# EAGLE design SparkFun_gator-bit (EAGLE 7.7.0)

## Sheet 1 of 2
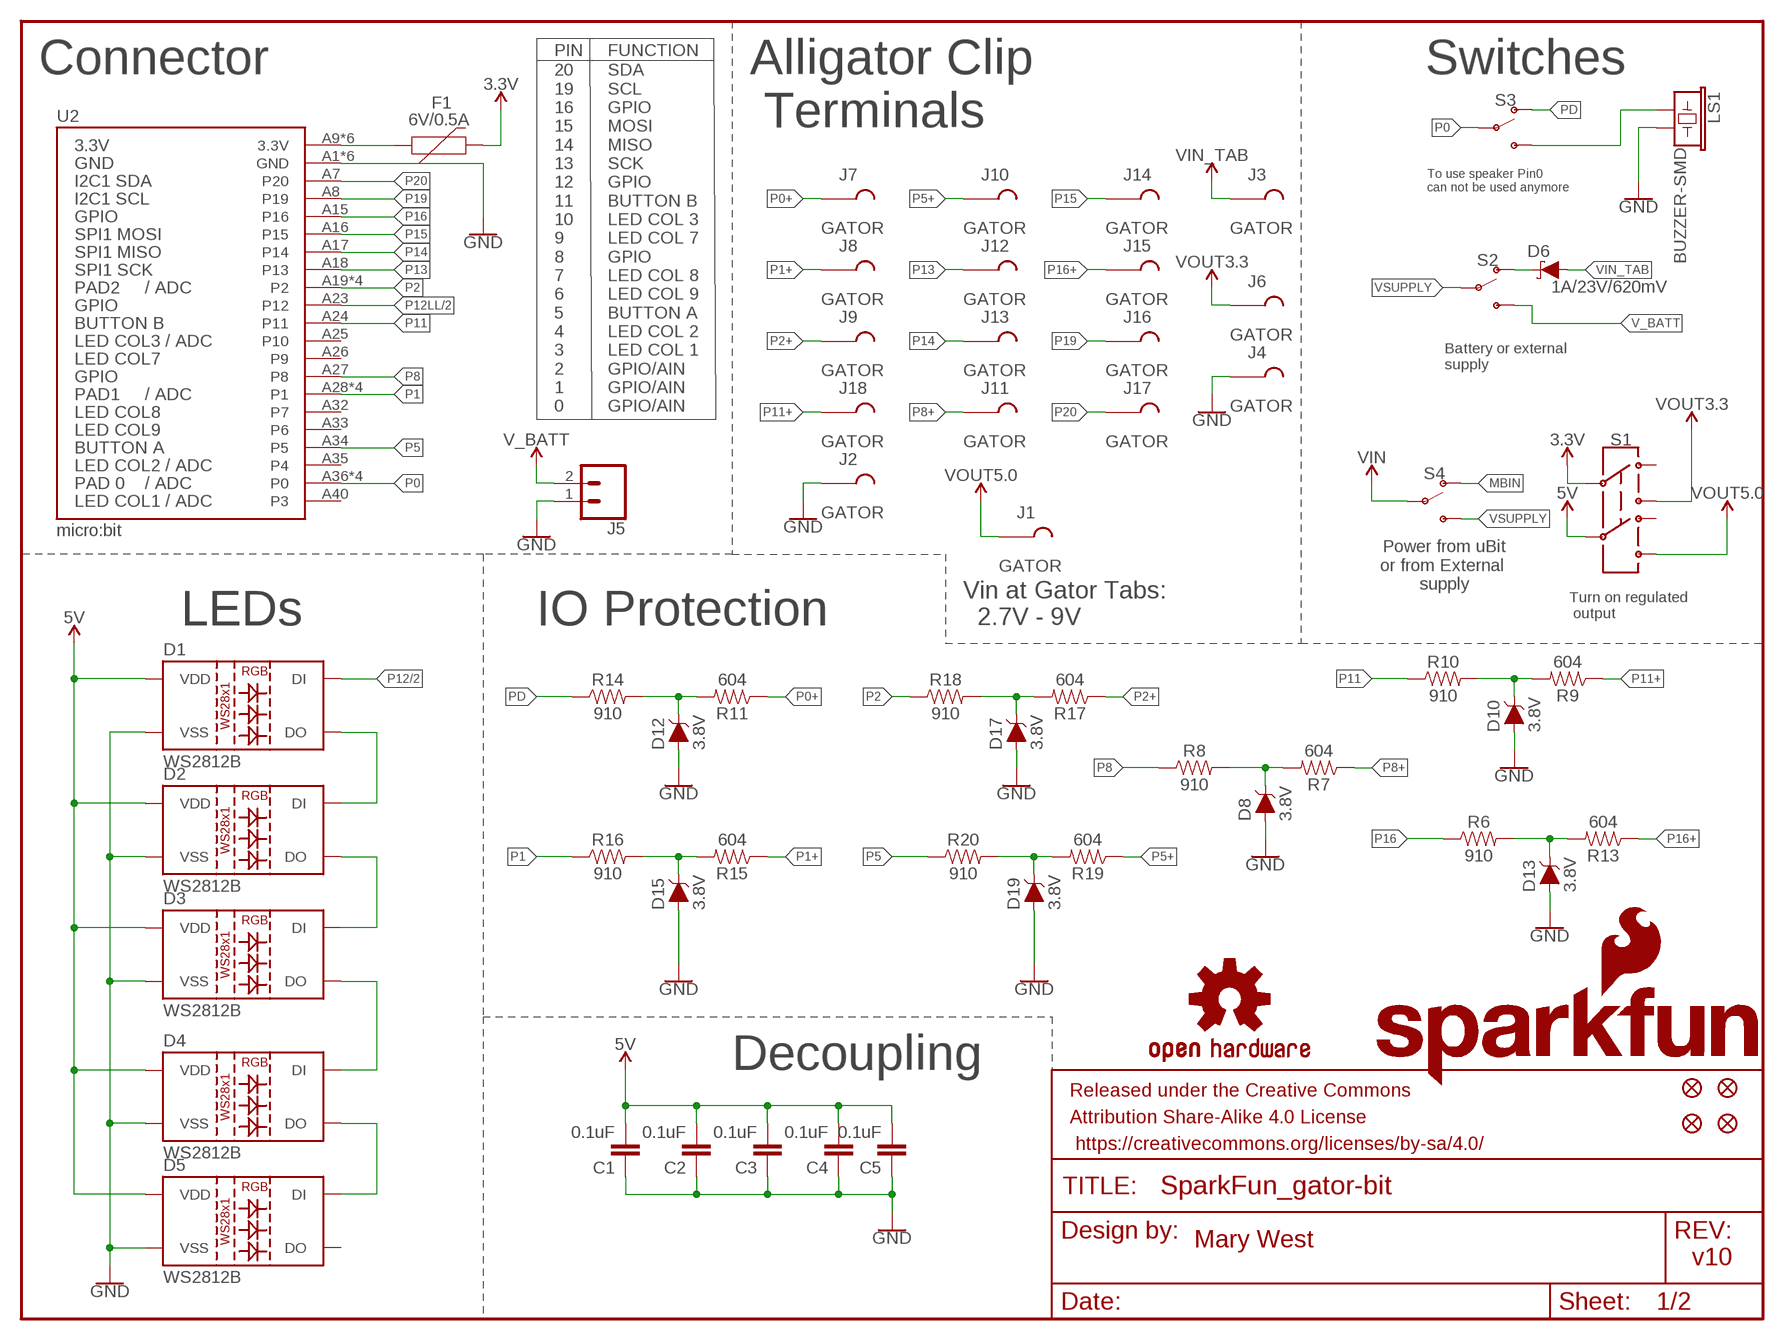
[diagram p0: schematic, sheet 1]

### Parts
C1  0.1uF  0.1UF-0603-25V-(+80/-20%)  [0603]
C2  0.1uF  0.1UF-0603-25V-(+80/-20%)  [0603]
C3  0.1uF  0.1UF-0603-25V-(+80/-20%)  [0603]
C4  0.1uF  0.1UF-0603-25V-(+80/-20%)  [0603]
C5  0.1uF  0.1UF-0603-25V-(+80/-20%)  [0603]
D1  WS2812B  [WS2812B]
D2  WS2812B  [WS2812B]
D3  WS2812B  [WS2812B]
D4  WS2812B  [WS2812B]
D5  WS2812B  [WS2812B]
D6  1A/23V/620mV  DIODE-SCHOTTKY-BAT20J  [SOD-323]
D8  3.8V  PDZVTR3.6B  [SOD-128]
D10  3.8V  PDZVTR3.6B  [SOD-128]
D12  3.8V  PDZVTR3.6B  [SOD-128]
D13  3.8V  PDZVTR3.6B  [SOD-128]
D15  3.8V  PDZVTR3.6B  [SOD-128]
D17  3.8V  PDZVTR3.6B  [SOD-128]
D19  3.8V  PDZVTR3.6B  [SOD-128]
F1  6V/0.5A  PPTC_HALF-AMP  [1206]
FD1  FIDUCIAL1X2  [FIDUCIAL-1X2]
FD2  FIDUCIAL1X2  [FIDUCIAL-1X2]
FD3  FIDUCIAL1X2  [FIDUCIAL-1X2]
FD4  FIDUCIAL1X2  [FIDUCIAL-1X2]
FRAME1  FRAME-LETTER  [CREATIVE_COMMONS]
J1  GATOR  [GATOR]
J2  GATOR  [GATOR]
J3  GATOR  [GATOR]
J4  GATOR  [GATOR]
J5  CONN_02-JST-2MM-SMT  [JST-2-SMD]
J6  GATOR  [GATOR]
J7  GATOR  [GATOR]
J8  GATOR  [GATOR]
J9  GATOR  [GATOR]
J10  GATOR  [GATOR]
J11  GATOR  [GATOR]
J12  GATOR  [GATOR]
J13  GATOR  [GATOR]
J14  GATOR  [GATOR]
J15  GATOR  [GATOR]
J16  GATOR  [GATOR]
J17  GATOR  [GATOR]
J18  GATOR  [GATOR]
LOGO1  SFE_LOGO_NAME_FLAME.3_INCH  [SFE_LOGO_NAME_FLAME_.3]
LOGO2  OSHW-LOGOM  [OSHW-LOGO-M]
LS1  BUZZER-SMD  [BUZZER-CCV]
R6  910  910OHMOHMS-0603-1/10W-1%  [0603]
R7  604  604OHMOHMS-0603-1/10W-1%  [0603]
R8  910  910OHMOHMS-0603-1/10W-1%  [0603]
R9  604  604OHMOHMS-0603-1/10W-1%  [0603]
R10  910  910OHMOHMS-0603-1/10W-1%  [0603]
R11  604  604OHMOHMS-0603-1/10W-1%  [0603]
R13  604  604OHMOHMS-0603-1/10W-1%  [0603]
R14  910  910OHMOHMS-0603-1/10W-1%  [0603]
R15  604  604OHMOHMS-0603-1/10W-1%  [0603]
R16  910  910OHMOHMS-0603-1/10W-1%  [0603]
R17  604  604OHMOHMS-0603-1/10W-1%  [0603]
R18  910  910OHMOHMS-0603-1/10W-1%  [0603]
R19  604  604OHMOHMS-0603-1/10W-1%  [0603]
R20  910  910OHMOHMS-0603-1/10W-1%  [0603]
S1  SWITCH-DPDT-SMD-AYZ0202  [SWITCH_DPDT_SMD_AYZ0202]
S2  SWITCH-SPDT-SMD-AYZ0202  [SWITCH_DPDT_SMD_AYZ0202]
S3  SWITCH-SPDT-SMD-AYZ0202  [SWITCH_DPDT_SMD_AYZ0202]
S4  SWITCH-SPDT-SMD-AYZ0202  [SWITCH_DPDT_SMD_AYZ0202]
U2  micro:bit  MICRO:BITLEDS_UP  [MICRO:BIT_RA_PTH]

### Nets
3.3V: F1.2 S1.2 ; also sheet 2
5V: C1.2 C2.2 C3.2 C4.2 C5.2 D1.1(VDD) D2.1(VDD) D3.1(VDD) D4.1(VDD) D5.1(VDD) S1.5 ; also sheet 2
GND: C1.1 C2.1 C3.1 C4.1 C5.1 D1.3(VSS) D2.3(VSS) D3.3(VSS) D4.3(VSS) D5.3(VSS) D8.P$2(A) D10.P$2(A) D12.P$2(A) D13.P$2(A) D15.P$2(A) D17.P$2(A) D19.P$2(A) J2.P$1 J2.P$2 J4.P$1 J4.P$2 J5.1 LS1.- U2.A1(GND) U2.A2(GND) U2.A3(GND) U2.A4(GND) U2.A5(GND) U2.A6(GND) ; also sheet 2
MBIN: F1.1 S4.1(O) U2.A9(3.3V) U2.A10(3.3V) U2.A11(3.3V) U2.A12(3.3V) U2.A13(3.3V) U2.A14(3.3V)
N$3: LS1.+ S3.3(S)
N$4: D1.2(DO) D2.4(DI)
N$5: D2.2(DO) D3.4(DI)
N$6: D3.2(DO) D4.4(DI)
N$7: D4.2(DO) D5.4(DI)
N$20: D6.C S2.1(O)
P0: S3.2(P) U2.A36(P0) U2.A37(P0) U2.A38(P0) U2.A39(P0)
P0+: J7.P$1 J7.P$2 R11.1
P1: R16.1 U2.A28(P1) U2.A29(P1) U2.A30(P1) U2.A31(P1)
P1+: J8.P$1 J8.P$2 R15.1
P2: R18.1 U2.A19(P2) U2.A20(P2) U2.A21(P2) U2.A22(P2)
P2+: J9.P$1 J9.P$2 R17.1
P5: R20.1 U2.A34(P5)
P5+: J10.P$1 J10.P$2 R19.1
P8: R8.1 U2.A27(P8)
P8+: J11.P$1 J11.P$2 R7.1
P11: R10.1 U2.A24(P11)
P11+: J18.P$1 J18.P$2 R9.1
P12: D1.4(DI) ; also sheet 2
P12LL: U2.A23(P12) ; also sheet 2
P13: J12.P$1 J12.P$2 U2.A18(P13)
P14: J13.P$1 J13.P$2 U2.A17(P14)
P15: J14.P$1 J14.P$2 U2.A16(P15)
P16: R6.1 U2.A15(P16)
P16+: J15.P$1 J15.P$2 R13.1
P19: J16.P$1 J16.P$2 U2.A8(P19)
P20: J17.P$1 J17.P$2 U2.A7(P20)
PD: R14.1 S3.1(O)
PP0: D12.P$1(C) R11.2 R14.2
PP1: D15.P$1(C) R15.2 R16.2
PP2: D17.P$1(C) R17.2 R18.2
PP5: D19.P$1(C) R19.2 R20.2
PP8: D8.P$1(C) R7.2 R8.2
PP11: D10.P$1(C) R9.2 R10.2
PP16: D13.P$1(C) R6.2 R13.2
V_BATT: J5.2 S2.3(S)
VIN: S4.2(P) ; also sheet 2
VIN_TAB: D6.A J3.P$1 J3.P$2
VOUT3.3: J6.P$1 J6.P$2 S1.3 ; also sheet 2
VOUT5.0: J1.P$1 J1.P$2 S1.6 ; also sheet 2
VSUPPLY: S2.2(P) S4.3(S)
Unconnected: D5.2(DO) S1.1 S1.4 U2.A25(P10) U2.A26(P9) U2.A32(P7) U2.A33(P6) U2.A35(P4) U2.A40(P3)

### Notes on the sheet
- PIN | FUNCTION
- Connector | Switches
- Alligator Clip
   Terminals
- To use speaker Pin0 
  can not be used anymore
- Battery or external
  supply
- 20
  19
  16
  15
  14
  13
  12
  11
  10
  9
  8
  7
  6
  5
  4
  3
  2
  1
  0
- SDA
  SCL
  GPIO
  MOSI
  MISO
  SCK
  GPIO
  BUTTON B
  LED COL 3
  LED COL 7
  GPIO
  LED COL 8
  LED COL 9
  BUTTON A
  LED COL 2
  LED COL 1
  GPIO/AIN
  GPIO/AIN
  GPIO/AIN
- Power from uBit
  or from External 
  supply
- Turn on regulated
   output
- LEDs | IO Protection
- Vin at Gator Tabs:
    2.7V - 9V
- Decoupling
- Mary West
- v10

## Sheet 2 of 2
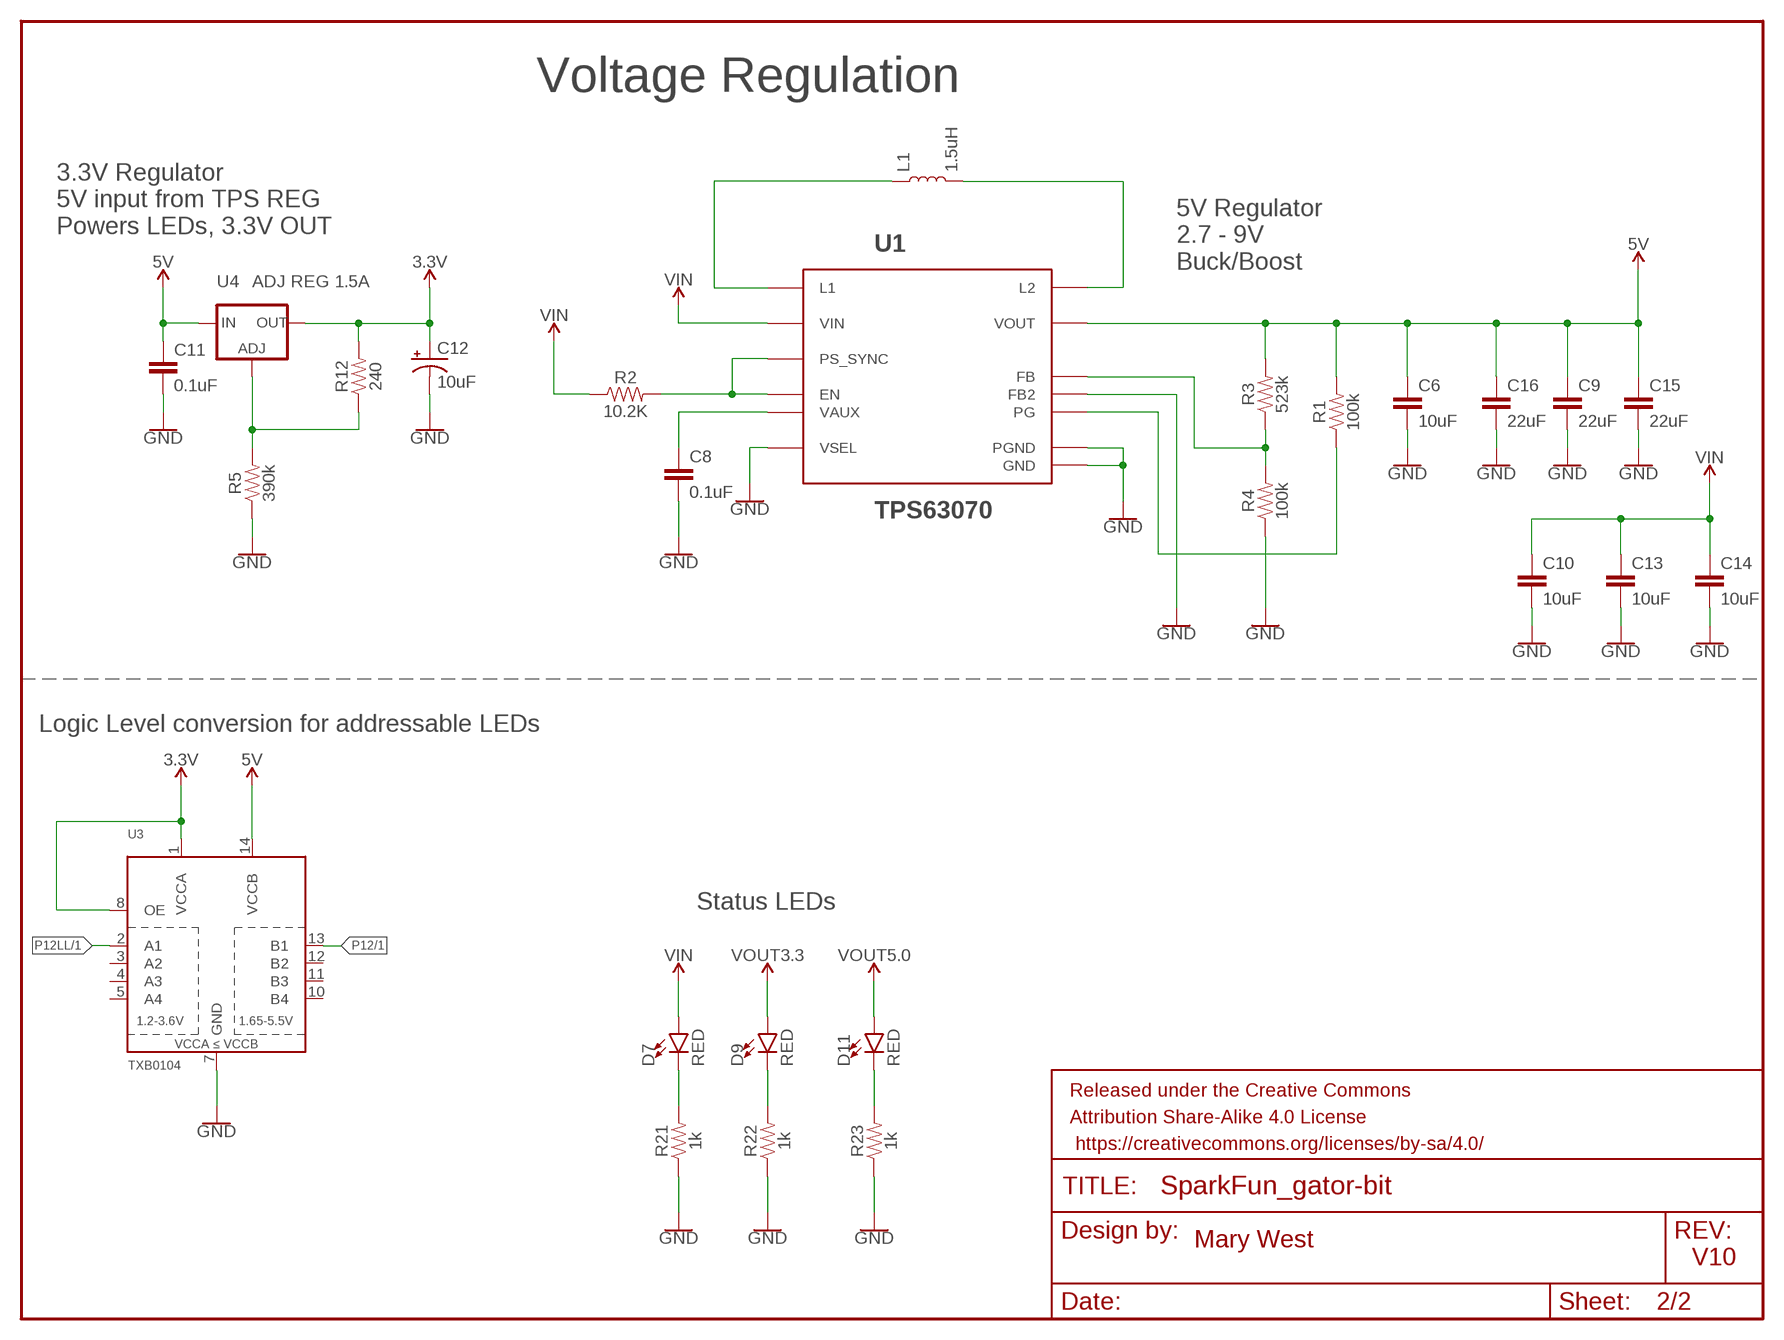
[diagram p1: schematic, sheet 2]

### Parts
C6  10uF  10UF-0603-6.3V-20%  [0603]
C8  0.1uF  0.1UF-0603-25V-(+80/-20%)  [0603]
C9  22uF  22UF-0805-6.3V-20%  [0805]
C10  10uF  10UF-0805-10V-10%  [0805]
C11  0.1uF  0.1UF-0603-25V-(+80/-20%)  [0603]
C12  10uF  10UF-POLAR-EIA3216-16V-10%(TANT)  [EIA3216]
C13  10uF  10UF-0805-10V-10%  [0805]
C14  10uF  10UF-0603-6.3V-20%  [0603]
C15  22uF  22UF-0805-6.3V-20%  [0805]
C16  22uF  22UF-0805-6.3V-20%  [0805]
D7  RED  LED-RED0603  [LED-0603]
D9  RED  LED-RED0603  [LED-0603]
D11  RED  LED-RED0603  [LED-0603]
FRAME3  FRAME-LETTER  [CREATIVE_COMMONS]
L1  1.5uH  INDUCTOR-XFL40201.5UH  [XFL4020]
R1  100k  100KOHM-0603-1/10W-1%  [0603]
R2  10.2K  10.2KOHM  [0603]
R3  523k  523KOHMOHMS-0603-1/10W-1%  [0603]
R4  100k  100KOHM-0603-1/10W-1%  [0603]
R5  390k  390KOHM-0603-1/10W-1%  [0603]
R12  240  240OHM-0603-1/10W-1%  [0603]
R21  1k  1KOHM-0603-1/10W-1%  [0603]
R22  1k  1KOHM-0603-1/10W-1%  [0603]
R23  1k  1KOHM-0603-1/10W-1%  [0603]
U1  TPS63070  TPS63070RNM  [TPS63070RNM]
U3  TXB0104  TXB0104PWR  [TSSOP14]
U4  ADJ REG 1.5A  GATORBIT_LM317  [SOT223]

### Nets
3.3V: C12.+ R12.2 U3.1(VCCA) U3.8(OE) U4.2(OUT) U4.4(OUT) ; also sheet 1
5V: C6.1 C9.1 C11.1 C15.1 C16.1 R1.2 R3.2 U1.P$7(VOUT) U3.14(VCCB) U4.3(IN) ; also sheet 1
GND: C6.2 C8.2 C9.2 C10.2 C11.2 C12.- C13.2 C14.2 C15.2 C16.2 R4.1 R5.1 R21.1 R22.1 R23.1 U1.P$4(GND) U1.P$6(FB2) U1.P$10(PGND) U1.P$15(VSEL) U3.7(GND) ; also sheet 1
N$2: L1.P$1 U1.P$11(L1)
N$8: L1.P$2 U1.P$9(L2)
N$9: D7.C R21.2
N$11: R3.1 R4.2 U1.P$5(FB)
N$12: C8.1 U1.P$3(VAUX)
N$13: R2.2 U1.P$1(PS_SYNC) U1.P$14(EN)
N$14: R1.1 U1.P$2(PG)
N$16: R5.2 R12.1 U4.1(ADJ)
N$23: D9.C R22.2
N$24: D11.C R23.2
P12: U3.13(B1) ; also sheet 1
P12LL: U3.2(A1) ; also sheet 1
VIN: C10.1 C13.1 C14.1 D7.A R2.1 U1.P$12(VIN) ; also sheet 1
VOUT3.3: D9.A ; also sheet 1
VOUT5.0: D11.A ; also sheet 1
Unconnected: U3.3(A2) U3.4(A3) U3.5(A4) U3.10(B4) U3.11(B3) U3.12(B2)

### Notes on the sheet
- Voltage Regulation
- 3.3V Regulator
  5V input from TPS REG
  Powers LEDs, 3.3V OUT
- 5V Regulator
  2.7 - 9V
  Buck/Boost
- Logic Level conversion for addressable LEDs
- Status LEDs
- Mary West
- V10

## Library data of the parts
C1-C5 C8 C11 = SparkFun-Capacitors:0.1UF: 0.1µF ceramic capacitors; PROD_ID: CAP-00810
C6 C14 = SparkFun-Capacitors:10UF: 10.0µF ceramic capacitors; PROD_ID: CAP-11015
C9 C15 C16 = SparkFun-Capacitors:22UF: 22µF ceramic capacitors; PROD_ID: CAP-08402
C10 C13 = SparkFun-Capacitors:10UF: 10.0µF ceramic capacitors; PROD_ID: CAP-11330
C12 = SparkFun-Capacitors:10UF-POLAR: 10.0µF polarized capacitors; PROD_ID: CAP-00811
D1-D5 = SparkFun-LED:WS2812B: WS2812B SMD addressable RGB LED 5x5mm SMD LED with built-in controller IC. Color: Red/Green/Blue mC Rating: RGB: 390, 660, 180 mcd Forward Voltage: RGB: 2.0, 3.0, 3.0 V Packages:WS2812B SparkFun Products: Blynk Board - ESP8266; PROD_ID: DIO-12503
D6 = SparkFun-DiscreteSemi:DIODE-SCHOTTKY: Schottky diode; PROD_ID: DIO-11623
D7 D9 D11 = SparkFun-LED:LED-RED: Red SMD LED; PROD_ID: DIO-00819
D8 D10 D12 D13 D15 D17 D19 = PDZVTR36BCT:PDZVTR3.6B: Zener Diode; PROD_ID: DIO-13895; TECHNOLOGIES: Zener Diode 3.8V 1W ±5.26% Surface Mount PMDTM
F1 = SparkFun-Fuses:PPTC: Resettable Fuse PPTC; PROD_ID: RES-08585
FD1-FD4 = SparkFun-Aesthetics:FIDUCIAL: Fiducial Alignment Points
FRAME1 FRAME3 = SparkFun-Aesthetics:FRAME-LETTER: Schematic Frame - Letter
J1-J4 J6-J18 = TAB:GATOR
J5 = SparkFun-Connectors:CONN_02: Multi connection point. Often used as Generic Header-pin footprint for 0.1 inch spaced/style header connections; PROD_ID: CONN-11443
L1 = SparkFun-Coils:INDUCTOR-XFL4020; PROD_ID: INDUC-13855
LOGO1 = SparkFun-Aesthetics:SFE_LOGO_NAME_FLAME: SparkFun Font Logo w/ Flame
LOGO2 = SparkFun-Aesthetics:OSHW-LOGO: Open-Source Hardware (OSHW) Logo
LS1 = SparkFun-Electromechanical:BUZZER: Buzzer; PROD_ID: COMP-08568
R1 R4 = SparkFun-Resistors:100KOHM: 100kΩ resistor; PROD_ID: RES-07828
R2 = SparkFun-Resistors:10.2KOHM: https://www.digikey.com/product-detail/en/yageo/RC0603FR-0710K2L/311-10.2KHRTR-ND/726883; PROD_ID: RES-13856
R3 = SparkFun-Resistors:523KOHM; PROD_ID: RES-13864
R5 = SparkFun-Resistors:390KOHM: 390kΩ resistor; PROD_ID: RES-12024
R6 R8 R10 R14 R16 R18 R20 = SparkFun-Resistors:910OHM: 910Ω resistor; PROD_ID: RES-13860
R7 R9 R11 R13 R15 R17 R19 = SparkFun-Resistors:604OHM; PROD_ID: RES-13857
R12 = SparkFun-Resistors:240OHM: 240Ω resistor; PROD_ID: RES-07849
R21-R23 = SparkFun-Resistors:1KOHM: 1kΩ resistor; PROD_ID: RES-07856
S1 = SparkFun-Switches:SWITCH-DPDT: Double-Pole, Double-Throw (DPDT) Switch Double-pole, double-throw switches. Variant Overview PTH-GPI-152-3013 Used on SparkFun Geiger Counter SMD-AY0202 Surface Mount DPDT Switch (COM-00597) Used on e.g. LilyPad Arduino USB - ATmega32U4 Board; PROD_ID: SWCH-08179; SF_SKU: COM-00597
S2-S4 = SparkFun-Switches:SWITCH-SPDT: Single Pole, Double Throw (SPDT) Switch Single-pole, double-throw (SPDT) switch. Variant Overview SMD-AYZ0202 Surface Mount DPDT Switch (COM-00597) Used on e.g. LilyPad Arduino USB - ATmega32U4 Board PTH-11.6X4.0MM SPDT Mini Power Switch (COM-00102) Used on e.g. SparkFun Simon Says - Through-Hole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; PROD_ID: SWCH-08179; SF_ID: COM-00597
U1 = SparkFun-IC-Power:TPS63070RNM: The TPS6307x is a high efficiency, low quiescent current buck-boost converter suitable for applications where the input voltage can be higher or lower than the output voltage. Output currents can go as high as 2 A in boost mode and in buck mode. The buck-boost converter is based on a fixed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; PROD_ID: IC-13858
U2 = Micro_Bit_Parts:MICRO:BIT: BBC MICRO_BIT with 5x5 LED array facing the direction noted in the variant. "UP" means away from the host board, "Down" means facing towards the host board.; PROD_ID: CONN-13452
U3 = SparkFun-IC-Comms:TXB0104PWR: 4-Bit Bi-Directional Level Shifter 1.2V-3.6V (VCCA) to 1.65V-5.5V (VCCB) bi-directional level shifter with auto direction sensing. Max data rate - VCCA 1.8V: 20Mbps (50ns), VCCA 3.3V: 100Mbps (10ns) Digikey: 296-21929-1-ND (TSSOP) Datasheet SparkFun Products SparkFun Cellular Shield - MG2639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; PROD_ID: IC-13929
U4 = SparkFun-IC-Power:GATORBIT_LM317; PROD_ID: VREG-12029

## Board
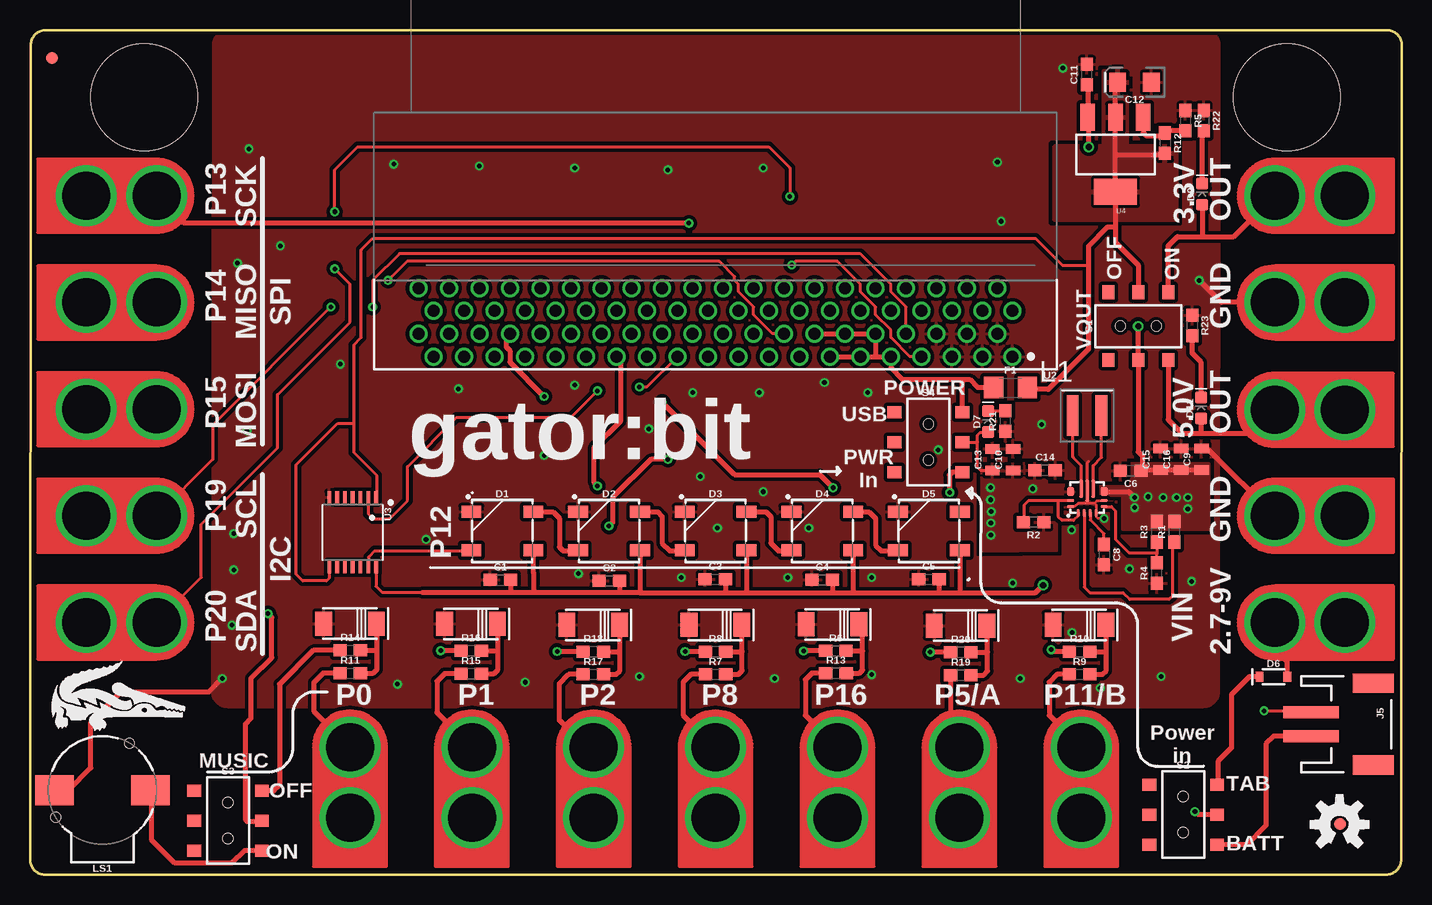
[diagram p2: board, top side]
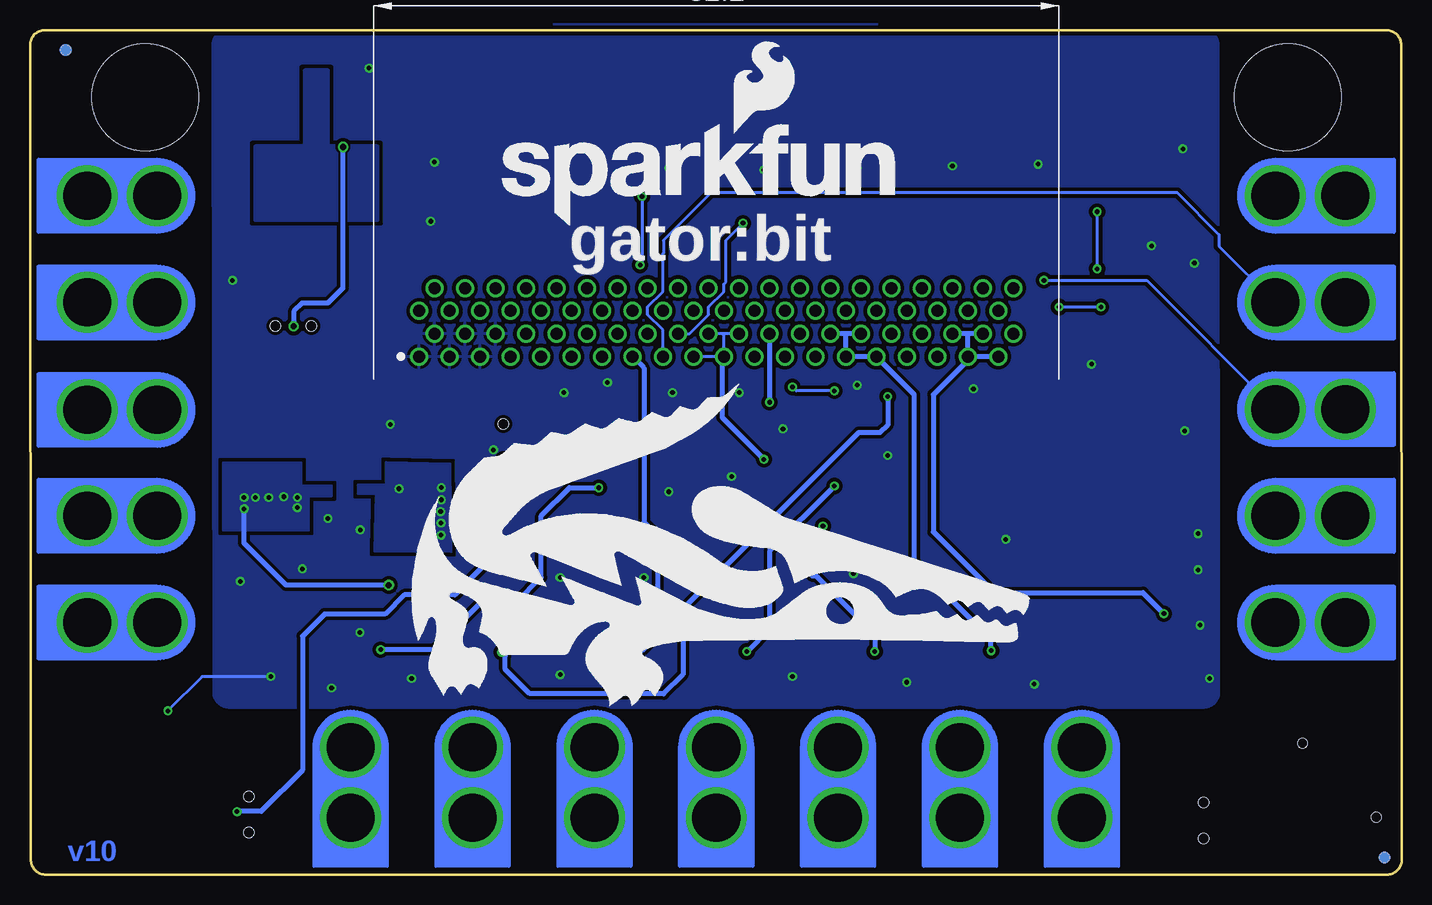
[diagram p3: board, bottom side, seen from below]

Size 114.36 x 70.39 mm. Coordinates in mm from the lower left corner, seen from the top.
Outline: 0.06,69.12 0,1.27 arc90 1.27,0 113.03,0 arc90 114.3,1.27 114.36,69.12 arc90 113.09,70.39 1.33,70.39 arc90 0.06,69.12
Copper layers (1*16): Top 0.035mm / dielectric 1.5mm / Bottom 0.035mm
Design rules "SparkFun-2-layer-TIGHT": minimum track width 7mil, minimum drill 15mil, track to track 7mil, track to pad 7mil, pad to pad 7mil, via to via 7mil, smd to smd 7mil, copper to edge 7mil, drill to drill 7mil, minimum pad ring 7mil, minimum via ring 7mil, stop-mask expansion 4mil, vias tented up to drill 25mil, thermal gap 10mil
Holes 8.89 mm at 9.53,64.77 104.77,64.77

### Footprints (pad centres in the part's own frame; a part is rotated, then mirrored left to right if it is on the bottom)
0603 = smd 1.1 x 1: 1 -0.85,0; 2 0.85,0
0805 = smd 0.8 x 1.2: 1 -0.9,0; 2 0.9,0
EIA3216 = smd 1.4 x 1.6: + 1.4,0; - -1.4,0
WS2812B = smd 1.651 x 1: 1 2.577,-1.6; 2 2.577,1.6; 3 -2.577,1.6; 4 -2.577,-1.6
SOD-323 = smd 0.63 x 0.83: A 1.15,0; C -1.15,0
LED-0603 = smd 1 x 1: A -0.877,0; C 0.877,0
SOD-128 = smd 2 x 1.4: P$1 0,2.5; P$2 0,-1.9
1206 = smd 1.6 x 1.8: 1 -1.4,0; 2 1.4,0
FIDUCIAL-1X2 = smd 1 x 1: 1 0,0
GATOR = drill 4 pad 5.08: P$1 0,-6.096; P$2 0,-0.254
JST-2-SMD = smd 1 x 4.6: 1 -1,-3.7; 2 1,-3.7 | smd 1.6 x 3.4: NC1 -3.4,1.5; NC2 3.4,1.5
XFL4020 = smd 0.98 x 3.4: P$1 1,1.8; P$2 3.4,1.8
BUZZER-CCV = smd 3.2 x 2.5: + 4,0; - -4,0 | hole 0.8: -3.9,-2.25; 2.25,3.9
SWITCH_DPDT_SMD_AYZ0202 = smd 1 x 1.15: 1 -2.5,2.825; 2 0,2.825; 3 2.5,2.825; 4 -2.5,-2.825; 5 0,-2.825; 6 2.5,-2.825 | hole 0.85: 1.5,0; -1.5,0
TPS63070RNM = smd 0.6 x 0.25: P$1 0,2.145; P$2 0,1.645; P$3 0,1.145; P$4 0,0.645 | smd 0.25 x 0.6: P$5 0.5,-0.005; P$6 1,-0.005; P$14 1,2.795; P$15 0.5,2.795 | smd 0.75 x 0.6: P$7 1.757,0.006; P$12 1.768,2.794 | smd 1.45 x 0.35: P$9 1.988,0.895; P$11 1.988,1.895 | smd 1.8 x 0.35: P$10 1.812,1.395
MICRO:BIT_RA_PTH = drill 1: A1 -24.765,7.62; A2 -23.495,5.72; A3 -22.225,7.62; A4 -20.955,5.72; A5 -19.685,7.62; A6 -18.415,5.72; A7 -17.145,7.62; A8 -15.875,5.72; A9 -14.605,7.62; A10 -13.335,5.72; A11 -12.065,7.62; A12 -10.795,5.72; A13 -9.525,7.62; A14 -8.255,5.72; A15 -6.985,7.62; A16 -5.715,5.72; A17 -4.445,7.62; A18 -3.175,5.72; A19 -1.905,7.62; A20 -0.635,5.72; A21 0.635,7.62; A22 1.905,5.72; A23 3.175,7.62; A24 4.445,5.72; A25 5.715,7.62; A26 6.985,5.72; A27 8.255,7.62; A28 9.525,5.72; A29 10.795,7.62; A30 12.065,5.72; A31 13.335,7.62; A32 14.605,5.72; A33 15.875,7.62; A34 17.145,5.72; A35 18.415,7.62; A36 19.685,5.72; A37 20.955,7.62; A38 22.225,5.72; A39 23.495,7.62; A40 24.765,5.72; B1 -24.765,3.82; B2 -23.495,1.92; B3 -22.225,3.82; B4 -20.955,1.92; B5 -19.685,3.82; B6 -18.415,1.92; B7 -17.145,3.82; B8 -15.875,1.92; B9 -14.605,3.82; B10 -13.335,1.92; B11 -12.065,3.82; B12 -10.795,1.92; B13 -9.525,3.82; B14 -8.255,1.92; B15 -6.985,3.82; B16 -5.715,1.92; B17 -4.445,3.82; B18 -3.175,1.92; B19 -1.905,3.82; B20 -0.635,1.92; B21 0.635,3.82; B22 1.905,1.92; B23 3.175,3.82; B24 4.445,1.92; B25 5.715,3.82; B26 6.985,1.92; B27 8.255,3.82; B28 9.525,1.92; B29 10.795,3.82; B30 12.065,1.92; B31 13.335,3.82; B32 14.605,1.92; B33 15.875,3.82; B34 17.145,1.92; B35 18.415,3.82; B36 19.685,1.92; B37 20.955,3.82; B38 22.225,1.92; B39 23.495,3.82; B40 24.765,1.92
TSSOP14 = smd 0.305 x 0.991: 1 -1.95,-2.918; 2 -1.3,-2.918; 3 -0.65,-2.918; 4 0,-2.918; 5 0.65,-2.918; 6 1.3,-2.918; 7 1.95,-2.918; 8 1.95,2.918; 9 1.3,2.918; 10 0.65,2.918; 11 0,2.918; 12 -0.65,2.918; 13 -1.3,2.918; 14 -1.95,2.918
SOT223 = smd 1.219 x 2.235: 1 -2.311,-3.099; 2 0,-3.099; 3 2.311,-3.099 | smd 3.6 x 2.2: 4 0,3.099

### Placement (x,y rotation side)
C1  39.22,24.56 0 top
C2  48.29,24.49 0 top
C3  57.13,24.62 0 top
C4  66.04,24.56 0 top
C5  74.93,24.62 0 top
C6  91.76,33.66 180 top
C8  89.53,26.67 270 top
C9  97.65,34.61 90 top
C10  81.95,34.58 90 top
C11  88.11,66.67 90 top
C12  92.07,66.04 180 top
C13  80.23,34.58 90 top
C14  84.61,33.72 0 top
C15  94.25,34.61 90 top
C16  95.96,34.61 90 top
D1  39.38,28.64 0 top
D2  48.27,28.64 0 top
D3  57.16,28.64 0 top
D4  66.04,28.64 0 top
D5  74.93,28.64 0 top
D6  103.66,16.51 0 top
D7  79.88,37.76 90 top
D8  56.83,20.82 270 top
D9  97.71,56.71 90 top
D10  87.19,20.82 270 top
D11  97.64,38.89 90 top
D12  26.38,20.92 270 top
D13  66.61,20.86 270 top
D15  36.46,20.89 270 top
D17  46.65,20.82 270 top
D19  77.28,20.76 270 top
F1  81.74,40.59 0 top
FD1  1.47,1.43 0 bottom
FD2  1.81,68.07 0 top
FD3  109.22,4.2 0 top
FD4  111.38,68.7 0 bottom
FRAME1  not placed on the board
FRAME3  not placed on the board
J1  103.5,38.73 90 top
J2  103.51,47.69 90 top
J3  103.51,21.02 90 top
J4  103.51,29.91 90 top
J5  110.49,12.54 270 top
J6  103.51,56.58 90 top
J7  26.68,10.86 0 top
J8  36.84,10.86 0 top
J9  46.99,10.86 0 top
J10  77.47,10.86 0 top
J11  57.16,10.86 0 top
J12  10.8,56.58 270 top
J13  10.8,47.69 270 top
J14  10.8,38.8 270 top
J15  67.31,10.86 0 top
J16  10.8,29.91 270 top
J17  10.8,21.02 270 top
J18  87.63,10.86 0 top
L1  85.92,36.46 0 top
LOGO1  75.56,53.98 0 bottom
LOGO2  109.16,4.19 0 top
LS1  6.04,7.04 0 top
R1  95.42,28.57 90 top
R2  83.66,29.37 180 top
R3  93.94,28.57 90 top
R4  93.94,25.13 90 top
R5  96.32,62.84 270 top
R6  67.18,18.64 0 top
R7  57.15,16.69 0 top
R8  57.15,18.59 0 top
R9  87.5,16.69 0 top
R10  87.5,18.59 0 top
R11  26.7,16.79 0 top
R12  94.61,60.96 270 top
R13  67.19,16.8 0 top
R14  26.7,18.69 0 top
R15  36.78,16.76 0 top
R16  36.78,18.67 0 top
R17  46.96,16.69 0 top
R18  46.96,18.59 0 top
R19  77.6,16.64 0 top
R20  77.6,18.54 0 top
R21  81.32,37.81 90 top
R22  97.84,62.84 270 top
R23  96.88,45.77 270 top
S1  92.39,45.72 0 top
S2  96.13,5 270 top
S3  16.52,4.5 270 top
S4  74.89,36.04 270 top
U1  89.53,30.16 90 top
U2  57.15,50.8 180 top
U3  26.9,28.52 180 top
U4  90.49,60.01 180 top
U$4  [ORDERING_INSTRUCTIONS]  not placed on the board

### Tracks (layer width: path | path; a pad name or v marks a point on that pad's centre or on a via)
3.3V
  Top 0.254: 88.26,50.8 86.04,50.8 83.82,53.02 28.57,53.02 27.62,52.07 27.62,44.77 26.99,44.13 26.99,37.72 | 26.99,37.72 26.99,35.19 28.88,33.3 28.88,31.47 U3.1 | U3.8 24.95,24.72 24.71,24.49 22.73,24.49 22.2,25.02 22.2,34.16 25.65,37.62 26.89,37.62 26.99,37.72
  Top 0.406: 90.49,53.98 U4.4 90.49,60.01 | 90.49,53.98 90.49,52.7 92.39,50.8 S1.2 | 90.49,53.98 89.85,53.98 88.26,52.39 88.26,50.8 88.26,43.81 84.89,40.44 83.29,40.44 F1.2 | C12.+ 90.49,65.85 U4.2 90.49,60.01 | 90.49,60.01 94.51,60.01 R12.2
  pour Top (isolate 0.305): 89.53,66.99 89.53,60.64 85.41,60.64 85.41,54.61 95.57,54.61 95.57,60.64 91.44,60.64 91.44,66.99
5V  (via drill 0.38, 0.51)
  Top 0.254: U3.14 28.85,24.03 29.36,23.52 33.38,23.52 33.4,23.5
  Top 0.406: C11.1 88.18,65.75 U4.3 88.26,63.02 v88.26,60.64 | 50.8,23.5 58.1,23.5 | 58.1,23.5 59.69,23.5 | 59.69,23.5 66.99,23.5 | 66.99,23.5 68.58,23.5 | 68.58,23.5 75.88,23.5 | 75.88,23.5 77.47,23.5 | 77.47,23.5 83.82,23.5 v84.45,24.13 | D1.1 41.95,25.18 41.96,25.18 41.96,23.5 | D2.1 50.84,23.54 50.8,23.5 | 58.1,23.5 57.98,23.62 C3.2 | D3.1 59.73,23.54 59.69,23.5 | C4.2 66.89,23.59 66.99,23.5 | D4.1 68.62,23.54 68.58,23.5 | C5.2 75.78,23.59 75.88,23.5 | D5.1 77.51,23.54 77.47,23.5 | C9.1 C16.1 C15.1 92.66,33.71 C6.1 92.71,33.76 92.71,34.92 92.39,35.24 S1.5 92.39,45.69 v92.38,45.71 | U1.P$7 91.59,31.92 v92.07,31.43 | 50.8,23.5 49.1,23.5 | 49.1,23.5 41.96,23.5 | 41.96,23.5 40.13,23.5 | 40.13,23.5 33.4,23.5 32.7,23.5 | C1.2 40.07,23.55 40.13,23.5 | C2.2 49.14,23.54 49.1,23.5
  Bottom 0.406: v84.45,24.13 93.03,24.13 96.52,27.62 v96.52,30.48 | v88.26,60.64 88.26,48.9 89.53,47.62 91.69,47.62 92.38,46.93 v92.38,45.71
  other vias: 95.57,31.43 94.46,31.43 93.21,31.5 96.52,31.43 92.09,30.58
  pour Top (isolate 0.305, no thermals): 89.22,32.38 91.76,32.38 91.76,34.29 98.27,34.29 98.27,28.73 91.12,28.73 91.12,31.59 89.22,31.59
  pour Bottom: 91.12,28.73 91.12,31.59 89.22,31.59 89.22,32.38 91.76,32.38 91.76,34.29 98.27,34.29 98.27,28.73
GND  (via drill 0.38)
  Top 0.203: 88.73,30.93 88.96,31.16 U1.P$6 | 88.73,30.93 88.89,30.78 U1.P$4 88.89,29.86 88.9,29.84 88.9,29.81 89.02,29.69 v89.53,29.69 | U1.P$15 87.02,30.66 87.05,30.68 87.12,30.68 87.38,30.94 88.73,30.94 88.73,30.93
  Top 0.254: U1.P$10 88.14,34.32 88.26,34.45 | v102.87,13.65 106.04,13.65 106.36,13.34 106.58,13.34 J5.1
  Top 0.406: 97.63,49.37 99.32,47.69 J2.P$2 J2.P$1 109.54,47.75 | LS1.- 3.23,7.04 5.08,8.89 5.08,12.7 7.62,15.24 14.92,15.24 v16.03,16.35 | C9.2 98.16,35.51 J4.P$2 J4.P$1 109.54,29.97
  Bottom 0.254: v94.3,16.51 100.01,16.51 v102.87,13.65
  other vias: 97.47,49.53 16.99,25.4 16.83,20.8 30.64,15.88 41.27,16.03 50.8,16.51 62.07,16.35 57.31,28.89 16.99,28.42 18.26,60.48 17.3,50.96 20.87,52.41 42.86,34.92 37.47,59.05 45.4,58.9 53.18,58.74 69.85,40.16 61.12,58.9 45.4,40.8 51.59,37.15 61.12,31.91 84.33,37.53 18.1,36.99 80.64,59.37 86.11,67.21 80.96,54.45 86.84,28.73 75.72,35.4 81.91,24.29 91.65,25.49 70.17,16.67 82.55,16.35 55.88,33.18 64.93,28.89 30.32,59.21 25.88,42.55 60.8,40.16 55.24,40.16 86.87,20.18 96.84,24.45 89.22,15.56 35.72,40.48 66.23,41.01 70.17,24.77 63.18,24.77 54.29,24.77 45.72,25.08 33.02,27.94
  pour Top (isolate 0.305, rank 2): 15.24,15.24 15.3,69.12 arc-90 16.57,70.39 97.85,70.39 arc-90 99.12,69.12 99.06,15.24 arc-90 97.79,13.97 16.51,13.97 arc-90
  pour Bottom (isolate 0.305, rank 2): 15.24,15.24 15.3,69.12 arc-90 16.57,70.39 arc-3 97.85,70.39 arc-90 99.12,69.12 99.06,15.24 arc-90 97.79,13.97 16.51,13.97 arc-90
MBIN
  Top 0.406: U2.A13 U2.A11 70.48,43.18 | 70.48,43.18 U2.A9 71.75,42.23 72.71,41.27 77.9,41.27 | U2.A14 U2.A12 U2.A10 70.48,43.18 | S4.1 77.72,41.09 77.9,41.27 | 77.9,41.27 78.33,41.27 78.99,40.62 80.31,40.62 F1.1
N$2
  Top 0.254: U1.P$11 87.64,34.09 86.93,34.8 86.94,34.81 86.94,38.24 L1.P$1
N$3
  Top 0.406: S3.3 17.88,2 16.83,0.95 12.06,0.95 10.16,2.86 10.16,6.92 LS1.+
N$4
  Top 0.406: D1.2 43.58,30.23 44.13,29.69 44.13,27.3 44.45,26.99 46.04,26.99 46.2,26.83 45.89,26.83 D2.4
N$5
  Top 0.406: D2.2 52.31,30.23 52.7,29.84 52.7,27.62 53.34,26.99 54.53,26.99 D3.4
N$6
  Top 0.406: D3.2 61.36,30.23 61.75,29.84 61.75,27.62 62.39,26.99 63.42,26.99 D4.4
N$7
  Top 0.406: D4.2 69.94,30.23 70.48,29.69 70.48,27.46 70.96,26.99 72.31,26.99 D5.4
N$8
  Top 0.254: U1.P$9 88.64,34.09 89.33,34.78 89.33,38.25 L1.P$2
N$9
  Top 0.254: D7.C 81.31,38.64 R21.2
N$11
  Top 0.254: U1.P$5 90.15,30.66 90.49,30.32 90.49,27.94 91.6,26.83 93.87,26.83 93.95,26.75 | R3.1 93.95,27.71 93.95,26.75 | R4.2 93.94,26.73 93.95,26.75
N$12
  Top 0.254: U1.P$3 88.39,29.56 89.53,28.42 C8.1
N$13
  Top 0.254: U1.P$1 87.39,29.92 86.99,29.53 86.04,29.53 85.72,29.84 85.72,31.16 | U1.P$14 85.72,31.16 | 85.72,31.16 83.23,31.16 82.87,30.8 82.87,29.43 R2.2
N$14
  Top 0.254: U1.P$2 87.89,23.96 88.36,23.5 91.12,23.5 91.68,22.94 94.94,22.94 95.26,23.25 95.26,27.57 R1.1
N$16
  Top 0.406: U4.1 92.8,61.82 93.03,61.59 94.4,61.59 R12.1 94.79,61.99 R5.2
N$20
  Top 0.406: D6.C 101.65,16.51 100.15,15.01 100.15,10.57 99.03,9.45 99.03,7.59 S2.1
N$22
  pour Bottom: 89.53,66.99 91.44,66.99 91.44,60.64 95.57,60.64 95.57,54.61 85.41,54.61 85.41,60.64 89.53,60.64
N$23
  Top 0.406: D9.C 97.71,61.86 R22.2
N$24
  Top 0.406: D11.C 97.64,42.7 96.88,43.46 R23.2
P0  (via drill 0.38)
  Top 0.254: v19.84,21.75 19.84,21.59
  Top 0.406: v19.84,21.75 20.16,21.43 20.16,18.1 18.41,16.35 18.41,13.02 17.94,12.54 17.94,4.6 18.1,4.45 19.28,4.45 S3.2
  Bottom 0.406: U2.A38 36.19,45.08 | 36.19,45.08 U2.A36 | U2.A37 36.19,45.08 | U2.A39 U2.A37 | U2.A37 36.19,42.86 39.05,40.01 39.05,28.57 33.97,23.5 21.59,23.5 v19.84,21.75
P0+
  Top 0.406: J7.P$1 J7.P$2 23.65,13.63 23.65,16 24.43,16.79 R11.1
P1  (via drill 0.38)
  Top 0.406: R16.1 v34.24,18.67
  Bottom 0.406: U2.A30 46.35,45.08 | 46.35,45.08 U2.A28 | 46.35,45.08 U2.A29 U2.A31 40.64,40.01 40.64,26.02 34.24,19.62 v34.24,18.67
P1+
  Top 0.406: J8.P$1 J8.P$2 33.92,13.51 33.92,16.13 34.56,16.76 R15.1
P2  (via drill 0.38)
  Top 0.406: R18.1 v43.95,18.59 | v53.18,34.61 51.75,34.61 48.58,31.43 48.58,29.37 v48.26,29.05
  Bottom 0.254: U2.A22 56.67,45.08 | 56.67,45.08 U2.A20 | 56.67,43.18 U2.A19 | U2.A21 56.51,44.92 56.67,45.08
  Bottom 0.406: U2.A21 56.67,43.18 56.67,38.1 v53.18,34.61 | v48.26,29.05 49.21,28.1 49.21,24.92 48.85,24.92 43.92,19.99 43.92,18.62 v43.95,18.59
P2+
  Top 0.406: J9.P$1 J9.P$2 46.87,10.48 46.51,10.48 44.13,12.86 44.13,15.92 44.9,16.69 R17.1
P5  (via drill 0.38)
  Top 0.406: v42.86,39.85 40,42.7 40,43.66 39.69,43.97 39.69,44.61 40,44.93 U2.A34 | R20.1 v75.06,18.54
  Bottom 0.406: v75.06,18.54 74.74,18.22 74.74,17.11 72.71,15.08 65.88,15.08 65.86,15.06 61.54,15.06 59.94,16.66 59.94,22.17 45.29,36.83 43.5,36.83 42.86,37.47 v42.86,39.85
P5+
  Top 0.406: J10.P$1 J10.P$2 76.75,11.33 R19.1
P8  (via drill 0.38)
  Top 0.406: U2.A27 49.21,42.86 49.21,37.78 46.99,35.56 46.99,32.7 v47.31,32.38 | R8.1 v54.61,18.59
  Bottom 0.406: v54.61,18.59 52.7,20.5 52.7,26.99 v47.31,32.38
P8+
  Top 0.406: J11.P$1 J11.P$2 54.45,13.3 54.45,16.05 55.09,16.69 R7.1
P11  (via drill 0.38)
  Top 0.406: v52.7,39.37 58.74,33.34 65.85,33.34 v66.94,32.24 | R10.1 85.28,18.59 v85.12,18.75
  Bottom 0.406: U2.A24 v52.7,39.37 | v66.94,32.24 66.95,32.26 69.39,32.26 71.75,29.9 71.75,24.77 73.82,22.7 76.76,22.7 80.72,18.75 v85.12,18.75
P11+
  Top 0.406: J18.P$1 J18.P$2 84.96,13.27 84.96,16.05 85.6,16.69 R9.1
P12
  Top 0.254: D1.4 36.75,26.99 28.74,26.99 28.22,26.47 28.22,25.63 U3.13
P12LL  (via drill 0.38)
  Top 0.254: v47.31,40.32 45.08,38.1 35.56,38.1 31.47,34.01 31.47,31.17 29.97,29.67 28.6,29.67 28.2,30.07 U3.2 | v50.8,40.64 51.43,40.64 U2.A23
  Bottom 0.254: v47.31,40.32 50.48,40.32 v50.8,40.64
P13  (via drill 0.38)
  Top 0.406: v54.93,54.29 12.83,54.29 J12.P$2
  Bottom 0.254: U2.A18 59.38,45.08 57.78,46.67 57.78,47.31 56.51,48.58 56.51,49.21 56.36,49.37 56.36,52.86 v54.93,54.29
  Bottom 0.406: J12.P$1 J12.P$2
P14
  Bottom 0.254: U2.A17 61.59,45.4 62.86,46.67 62.86,47.31 61.59,48.58 61.59,51.75 61.57,51.78 61.57,52.86 57.59,56.83 18.73,56.83 15.24,53.34 15.24,52.38 J13.P$2
  Bottom 0.406: J13.P$1 J13.P$2
P15  (via drill 0.38)
  Top 0.254: U2.A16 61.91,45.09 60.32,46.67 60.32,47.31 59.05,48.58 59.05,49.21 58.74,49.53 58.74,49.85 57.47,51.12 31.43,51.12 v29.84,49.53
  Bottom 0.254: v29.84,49.53 21.27,49.53 21.27,49.52 J14.P$2
  Bottom 0.406: J14.P$1 J14.P$2
P16  (via drill 0.38)
  Top 0.406: R6.1 v64.48,18.64
  Bottom 0.406: U2.A15 63.18,42.23 63.18,29.37 62.07,28.26 62.07,19.95 63.35,18.67 64.46,18.67 v64.48,18.64
P16+
  Top 0.406: J15.P$1 J15.P$2 64.64,13.27 64.64,16.26 65.18,16.8 R13.1
P19  (via drill 0.38)
  Top 0.254: U2.A8 73.02,47.31 71.75,48.58 71.75,49.21 69.21,51.75 30.8,51.75 28.57,49.53 v28.57,47.31 | v25.08,47.31 15.24,37.47 15.24,34.6 J16.P$2
  Top 0.406: J16.P$1 J16.P$2
  Bottom 0.254: v28.57,47.31 v25.08,47.31
P20  (via drill 0.38)
  Top 0.254: v25.4,50.48 26.67,49.21 26.67,46.04 20.64,40.01 20.64,35.56 14.29,29.21 14.29,24.77 J17.P$2 | v63.5,50.8 63.82,51.12 67.31,51.12 69.21,49.21 69.21,48.58 70.48,47.31 70.48,46.67 71.75,45.4 71.75,44.77 73.34,43.18 U2.A7 | v25.4,55.24 25.4,58.74 27.3,60.64 61.59,60.64 63.34,58.9 v63.34,56.52
  Bottom 0.254: v25.4,50.48 v25.4,55.24 | v63.34,56.52 63.34,50.96 v63.5,50.8
  Bottom 0.406: J17.P$1 9.78,21.02 10.16,20.64 10.17,20.64 J17.P$2
PD
  Top 0.406: S3.1 19.36,6.99 20.32,6.99 20.8,7.46 20.8,15.88 23.62,18.69 R14.1
PP0
  Top 0.406: R11.2 28.6,16.79 28.92,17.11 28.92,18.69 | 28.92,18.69 28.92,20.88 D12.P$1 | R14.2 28.92,18.69
PP1
  Top 0.406: R15.2 38.68,16.76 39,17.08 39,18.67 | 39,18.67 39,20.85 D15.P$1 | R16.2 39,18.67
PP2
  Top 0.406: R17.2 48.87,16.69 49.19,17 49.19,18.59 | 49.19,18.59 49.19,20.77 D17.P$1 | R18.2 49.19,18.59
PP5
  Top 0.406: R19.2 79.5,16.64 79.82,16.95 79.82,18.54 | 79.82,18.54 79.82,20.72 D19.P$1 | R20.2 79.82,18.54
PP8
  Top 0.406: R7.2 59.05,16.69 59.37,17 59.37,18.59 | 59.37,18.59 59.37,20.77 D8.P$1 | R8.2 59.37,18.59
PP11
  Top 0.406: R9.2 89.41,16.69 89.73,17 89.73,18.59 | 89.73,18.59 89.73,20.77 D10.P$1 | R10.2 89.73,18.59
PP16
  Top 0.406: R13.2 69.15,16.8 69.41,17.06 69.41,18.64 | 69.41,18.64 69.41,20.56 D13.P$1 | R6.2 69.41,18.64
V_BATT
  Top 0.406: J5.2 103.67,11.54 103.02,10.9 103.02,4.12 101.42,2.52 98.96,2.52 S2.3
VIN  (via drill 0.38)
  Top 0.254: 86.74,32.1 86.91,31.93 86.74,31.76 86.74,31.68 | 79.79,36.8 D7.A 79.86,36.86 79.22,36.86 78.99,36.64 78.99,36.04 | 78.99,36.04 78.99,33.94 79.26,33.68 C13.1 | S4.2 78.99,36.04
  other vias: 80.07,32.26 80.07,31.24 80.14,30.26 80.11,29.31 80.11,28.29 83.6,32.16
  pour Top (isolate 0.305): 79.34,34.23 84.68,34.32 84.71,32.48 84.93,32.48 86.99,32.51 86.99,31.59 86.04,31.59 85.57,31.11 85.57,26.99 79.34,26.92
  pour Bottom (isolate 0.305): 79.33,34.26 84.68,34.35 84.68,32.51 86.99,32.51 86.99,31.75 85.5,31.73 85.61,26.95 79.26,26.92
VIN_TAB
  Top 0.406: J3.P$1 J3.P$2 103.76,18.79 104.77,17.78 104.77,16.55 D6.A
VOUT3.3
  Top 0.254: J6.P$2 J6.P$1
  Top 0.406: S1.3 94.89,52.4 95.66,53.16 97.79,53.16 | 103.51,56.83 J6.P$2 | J6.P$2 103.76,53.92 | 97.79,53.16 100.35,53.16 J6.P$2 | D9.A 97.71,53.24 97.79,53.16
VOUT5.0
  Top 0.406: S1.6 94.89,37.92 96.01,36.8 97.61,36.8 | J1.P$2 J1.P$1 | J1.P$2 103.76,36.45 | D11.A 97.62,38.02 97.62,36.82 97.61,36.8 | 97.61,36.8 101.83,36.8 J1.P$2
VSUPPLY  (via drill 0.38)
  Top 0.406: v76.68,31.85 76.63,31.9 76.63,33.3 76.89,33.55 76.9,33.54 S4.3 | S2.2 97.36,5 v97.1,5.26
  Bottom 0.406: v76.68,31.85 76.66,31.83 76.66,25.6 78.94,23.32 83.16,23.32 84.76,21.72 89.81,21.72 91.64,19.89 91.64,8.71 95.07,5.28 97.08,5.28 v97.1,5.26

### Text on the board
Bottom: v10
tPlace: P13 | SCK | 3.3V | OUT | MISO | P14 | SPI | OFF | ON | GND | VOUT | P15 | MOSI | POWER | USB | OUT | 5.0V | gator:bit | PWR / In | P19 | SCL | I2C | GND | P12 | 2.7-9V | P20 | SDA | VIN | P0 | P1 | P2 | P8 | P16 | P5/A | P11/B | Power / in | MUSIC | OFF | TAB | ON | BATT
bPlace: gator:bit
Measures: * All dimensions / are in inches
tDocu: Mary West | Solder Mask: Black Gloss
